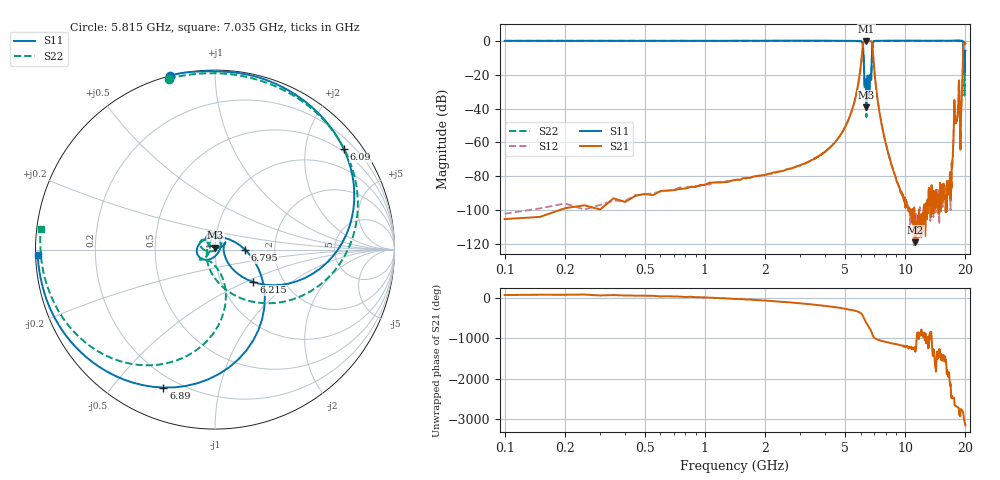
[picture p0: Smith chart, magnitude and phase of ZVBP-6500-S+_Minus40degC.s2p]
! Mini-Circuits
! S2P DATA File Format
! Type: BAND PASS FILTER
! Model: ZVBP-6500-S+
! All S Parameters are in dB deg format
! TEST CONDITIONS: INPUT POWER = 0 dBm @ Temperature = -40deg C
# MHZ S DB R 50
!Frequency  S11 dB  S11 DEG  S21 dB  S21 DEG  S12 dB  S12 DEG  S22 dB  S22 DEG
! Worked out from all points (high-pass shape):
!   1299 points, 100 MHz to 20 GHz, reference 50 ohm
!   highest |S21| = -0.12 dB at 6.405 GHz (marker M1); lowest = -119.1 dB at 11.25 GHz (marker M2)
!   |S21| within 3 dB of the highest: 6.154 GHz to 6.864 GHz (710.4 MHz wide, 10.9 % of centre); 19.53 GHz to end of sweep
!   lowest |S11| = -39.2 dB at 6.405 GHz (marker M3), VSWR 1.02, Z = 50.1 + j1.09 ohm
!   |S11| at or under -10 dB: 6.21 GHz to 6.816 GHz (606.9 MHz wide, 9.32 % of centre); 19.54888 GHz to 19.56711 GHz (18.23 MHz wide, 0.0932 % of centre); 19.74 GHz to 19.86 GHz (120 MHz wide, 0.606 % of centre)
!   |S22| runs from -45.0 to 0.0 dB; largest |S21 - S12| = 0.002
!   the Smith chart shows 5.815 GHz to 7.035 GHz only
!   S11 on the Smith chart (normalised r, x): 5.815 GHz: -0.00, +0.77; 6.09 GHz: 0.44, +2.85; 6.215 GHz: 1.42, -0.56; 6.795 GHz: 1.40, -0.00; 6.89 GHz: 0.15, -0.68; 7.035 GHz: 0.01, -0.02
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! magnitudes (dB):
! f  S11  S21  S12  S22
! 100 MHz  0.0  -105.3  -102.1  0.0
! 250 MHz  0.0  -97.1  -99.6  0.0
! 600 MHz  0.0  -88.7  -89.1  -0.1
! 1.45 GHz  0.0  -81.9  -82.2  0.0
! 3.45 GHz  0.1  -70.2  -70.2  0.0
! 4.875 GHz  0.0  -53.6  -53.6  -0.1
! 5.815 GHz  0.0  -26.4  -26.4  -0.1
! 6.09 GHz  -0.8  -8.1  -8.1  -0.9
! 6.215 GHz  -11.0  -0.5  -0.5  -11.2
! 6.405 GHz  -39.2  -0.1  -0.1  -45.0
! 6.49 GHz  -21.0  -0.2  -0.2  -21.3
! 6.62 GHz  -32.5  -0.1  -0.1  -30.6
! 6.795 GHz  -15.5  -0.3  -0.3  -15.3
! 6.89 GHz  -1.7  -5.4  -5.4  -1.8
! 7.035 GHz  -0.1  -18.8  -18.8  -0.2
! 8.275 GHz  0.1  -67.2  -67.2  -0.1
! 11.25 GHz  0.1  -119.1  -114.7  0.0
! 16.75 GHz  0.0  -77.6  -77.4  -0.1
! 17.75 GHz  0.2  -46.0  -45.9  -0.1
! 19 GHz  0.1  -46.2  -46.2  -0.1
! 19.6 GHz  -9.6  -1.3  -1.3  -10.2
! 20 GHz  -5.8  -1.8  -1.7  -6.2
